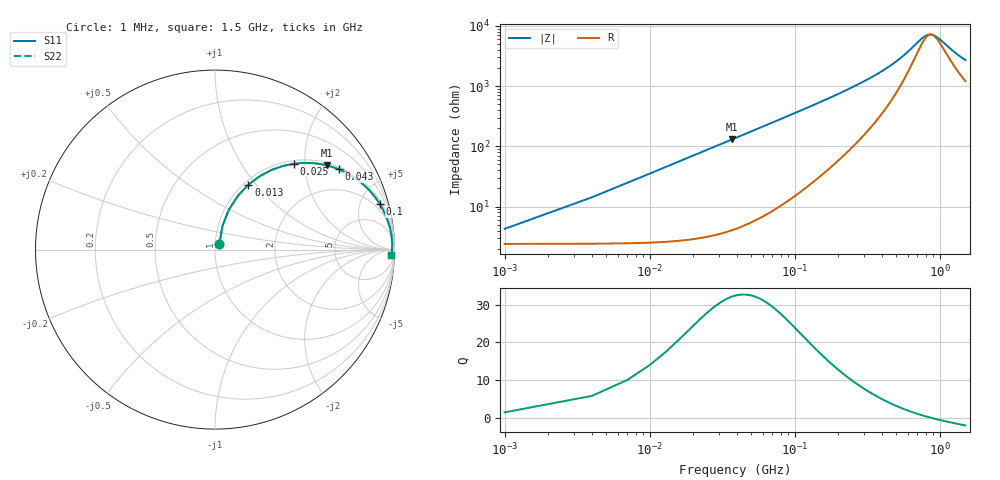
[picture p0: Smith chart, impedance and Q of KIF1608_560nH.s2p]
# MHz S RI R 50
!Freq ReS11 ImS11 ReS21 ImS21 ReS12 ImS12 ReS22 ImS22
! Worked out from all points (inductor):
!   501 points, 1 MHz to 1.5 GHz, reference 50 ohm
!   read as one part in series: L = 559 nH near 7 MHz
!   highest Q = 32.1 at 37 MHz (marker M1), where L = 560 nH
!   self-resonance near 873.4 MHz
!   S11 on the Smith chart (normalised r, x): 1 MHz: 1.05, +0.07; 13 MHz: 1.05, +0.91; 25 MHz: 1.06, +1.76; 43 MHz: 1.09, +3.03; 100 MHz: 1.30, +7.12; 1.5 GHz: 25, -48
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1  0.0246 0.0335  0.9754 -0.0335  0.9754 -0.0335  0.0246 0.0335
4  0.0416 0.1315  0.9584 -0.1315  0.9584 -0.1315  0.0416 0.1315
10  0.1271 0.2992  0.8729 -0.2992  0.8729 -0.2992  0.1271 0.2992
13  0.1866 0.3622  0.8134 -0.3622  0.8134 -0.3622  0.1866 0.3622
19  0.3161 0.4442  0.6839 -0.4442  0.6839 -0.4442  0.3161 0.4442
25  0.4385 0.4786  0.5615 -0.4786  0.5615 -0.4786  0.4385 0.4786
37  0.6256 0.4687  0.3744 -0.4687  0.3744 -0.4687  0.6256 0.4687
43  0.6913 0.4469  0.3087 -0.4469  0.3087 -0.4469  0.6913 0.4469
55  0.7831 0.3968  0.2169 -0.3968  0.2169 -0.3968  0.7831 0.3968
67  0.8407 0.3497  0.1593 -0.3497  0.1593 -0.3497  0.8407 0.3497
100  0.9179 0.2543  0.0821 -0.2543  0.0821 -0.2543  0.9179 0.2543
166  0.9639 0.1569  0.0361 -0.1569  0.0361 -0.1569  0.9639 0.1569
253  0.9795 0.099  0.0205 -0.099  0.0205 -0.099  0.9795 0.099
349  0.9848 0.0657  0.0152 -0.0657  0.0152 -0.0657  0.9848 0.0657
502  0.9871 0.0359  0.0129 -0.0359  0.0129 -0.0359  0.9871 0.0359
751  0.9869 0.00911  0.0131 -0.00911  0.0131 -0.00911  0.9869 0.00911
811  0.9866 0.00443  0.0134 -0.00443  0.0134 -0.00443  0.9866 0.00443
865  0.9863 0.000573  0.0137 -0.000573  0.0137 -0.000573  0.9863 0.000573
922  0.986 -0.0032  0.014 0.0032  0.014 0.0032  0.986 -0.0032
1003  0.9855 -0.00813  0.0145 0.00813  0.0145 0.00813  0.9855 -0.00813
1252  0.9841 -0.0211  0.0159 0.0211  0.0159 0.0211  0.9841 -0.0211
1500  0.9827 -0.032  0.0173 0.032  0.0173 0.032  0.9827 -0.032
